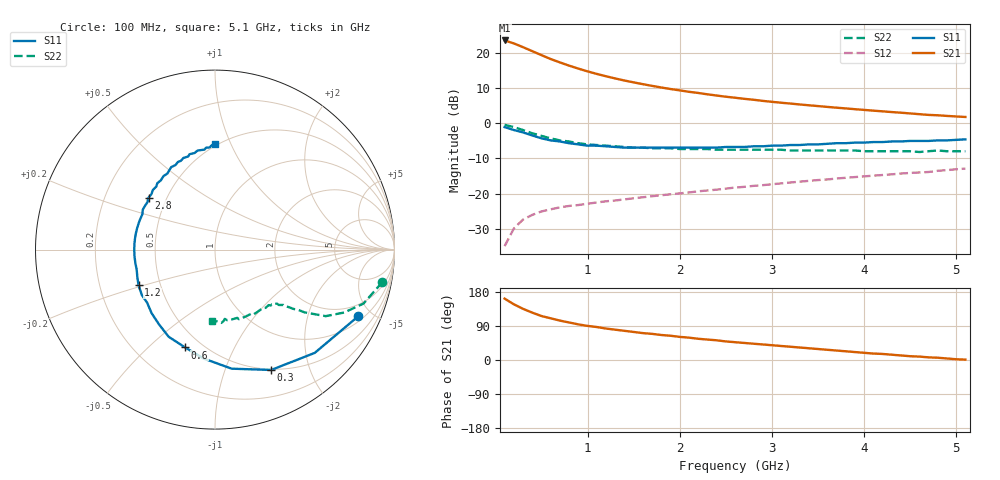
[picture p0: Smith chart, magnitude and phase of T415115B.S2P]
!AT-41511
!S-PARAMETERS at Vce=5V  Ic=5mA.  LAST UPDATED 01-25-95
# ghz s ma r 50
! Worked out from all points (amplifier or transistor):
!   51 points, 100 MHz to 5.1 GHz, reference 50 ohm
!   highest |S21| = 23.5 dB at 100 MHz (marker M1)
!   |S21| within 3 dB of that: start of sweep to 397 MHz
!   unconditionally stable (mu >= 1): 1.684 GHz to 4.755 GHz
!   at 900 MHz: K = 0.70, MSG = 19.4 dB, |S12| = -23.2 dB
!   at 2.6 GHz: K = 1.11, MAG = 10.8 dB, |S12| = -18.3 dB
!   at 5.1 GHz: K = 0.95, MSG = 7.3 dB, |S12| = -12.9 dB
!   lowest NFmin = 0.80 dB at 100 MHz
!   S11 on the Smith chart (normalised r, x): 100 MHz: 1.26, -4.15; 300 MHz: 0.49, -1.45; 600 MHz: 0.41, -0.66; 1.2 GHz: 0.38, -0.19; 2.8 GHz: 0.40, +0.30; 5.1 GHz: 0.48, +0.88
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0.1  0.88 -25.0  14.92 162.0  0.018 77.0  0.95 -11.0
0.2  0.8 -46.0  13.55 147.0  0.032 66.0  0.88 -20.0
0.3  0.74 -65.0  11.98 135.0  0.043 58.0  0.8 -26.0
0.4  0.67 -82.0  10.52 125.0  0.05 53.0  0.72 -31.0
0.5  0.61 -96.0  9.234 116.0  0.056 49.0  0.66 -33.0
0.6  0.57 -107.0  8.131 110.0  0.06 47.0  0.61 -35.0
0.7  0.55 -118.0  7.282 104.0  0.064 45.0  0.57 -36.0
0.8  0.52 -127.0  6.552 99.0  0.067 44.0  0.55 -37.0
0.9  0.5 -135.0  5.948 94.0  0.069 44.0  0.52 -38.0
1  0.48 -142.0  5.433 90.0  0.072 43.0  0.5 -39.0
1.2  0.47 -155.0  4.632 83.0  0.078 43.0  0.48 -40.0
1.4  0.45 -166.0  4.031 77.0  0.083 44.0  0.46 -41.0
1.5  0.45 -170.0  3.796 74.0  0.086 44.0  0.45 -42.0
1.6  0.45 -175.0  3.577 71.0  0.089 45.0  0.45 -43.0
1.8  0.45 176.0  3.21 66.0  0.095 45.0  0.44 -44.0
2.2  0.45 161.0  2.686 56.0  0.108 46.0  0.43 -48.0
2.6  0.46 148.0  2.298 47.0  0.122 46.0  0.42 -53.0
2.8  0.47 142.0  2.151 43.0  0.129 46.0  0.42 -55.0
3.5  0.5 122.0  1.749 29.0  0.156 45.0  0.41 -64.0
4  0.53 111.0  1.544 19.0  0.176 43.0  0.4 -72.0
4.3  0.55 105.0  1.439 14.0  0.188 42.0  0.4 -77.0
5.1  0.59 90.0  1.225 1.0  0.227 38.0  0.4 -92.0
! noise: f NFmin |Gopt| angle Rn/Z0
0.1  0.8  0.46  5  0.3
0.9  1  0.39  60  0.22
1.8  1.4  0.34  130  0.13
2.4  1.7  0.39  173  0.09
